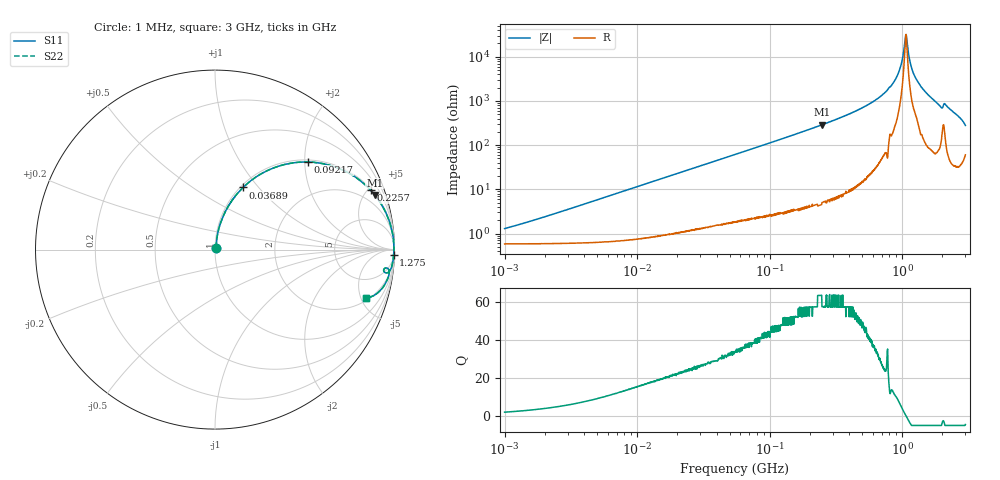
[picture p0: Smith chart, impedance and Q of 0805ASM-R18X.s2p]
!s-Parameter Generated by FASTRON Sdn. Bhd.
!FASTRON P/N : 0805ASM-R18X
!Keysight Technologies: E4991B_MY54100416_A.01.15
!Date: Fri Jun 19 14:50:46 2026
!Version  :Rev00  Fri Jun 19 14:50:46 2026
!Data & Calibration Information:
!Freq  S11  S21  S12  S22
!PortZ  Port1:50+j0  Port2:50+j0
!When reading reference impedance value at option line is always used.
! Remarks : This data is being provided solely for informational purposes.
# Hz S dB R 50
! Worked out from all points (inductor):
!   1601 points, 1 MHz to 3 GHz, reference 50 ohm
!   read as one part in series: L = 184 nH near 1.522 MHz
!   highest Q = 63.3 at 249.5 MHz (marker M1), where L = 185 nH
!   self-resonance near 1.065 GHz
!   S11 on the Smith chart (normalised r, x): 1 MHz: 1.01, +0.02; 36.89 MHz: 1.03, +0.83; 92.17 MHz: 1.05, +2.07; 225.7 MHz: 1.09, +5.20; 1.275 GHz: 10, -62; 3 GHz: 2.22, -5.47
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1000000  -37.80 62.6  -0.05 -0.7  -0.05 -0.7  -37.80 62.6
3804036  -27.10 79.6  -0.06 -2.5  -0.06 -2.5  -27.10 79.6
1.447069e7  -15.80 77.7  -0.19 -9.3  -0.19 -9.3  -15.80 77.7
3.688738e7  -8.41 65.7  -0.80 -22.3  -0.80 -22.3  -8.41 65.7
5.504702e7  -5.69 57.0  -1.52 -31.3  -1.52 -31.3  -5.69 57.0
9.216659e7  -2.97 43.4  -3.26 -45.2  -3.26 -45.2  -2.97 43.4
2.083556e8  -0.76 22.6  -8.32 -66.4  -8.32 -66.4  -0.76 22.6
2.257233e8  -0.65 20.9  -8.96 -68.1  -8.96 -68.1  -0.65 20.9
2.494827e8  -0.53 18.9  -9.80 -70.1  -9.80 -70.1  -0.53 18.9
5.284703e8  -0.10 7.4  -17.80 -81.3  -17.80 -81.3  -0.10 7.4
7.925923e8  -0.04 2.9  -25.90 -83.9  -25.90 -83.9  -0.04 2.9
9.395906e8  -0.03 1.3  -32.90 -81.3  -32.90 -81.3  -0.03 1.3
9.878038e8  -0.03 0.8  -37.00 -77.1  -37.00 -77.1  -0.03 0.8
1.0437e9  -0.03 0.2  -45.80 -53.1  -45.80 -53.1  -0.03 0.2
1.064802e9  -0.03 0.0  -50.00 -11.3  -50.00 -11.3  -0.03 0.0
1.097256e9  -0.03 -0.3  -44.90 55.8  -44.90 55.8  -0.03 -0.3
1.182785e9  -0.03 -1.1  -34.60 78.1  -34.60 78.1  -0.03 -1.1
1.274982e9  -0.04 -1.8  -30.00 80.2  -30.00 80.2  -0.04 -1.8
1.481494e9  -0.05 -3.4  -24.50 82.6  -24.50 82.6  -0.05 -3.4
1.912199e9  -0.18 -7.1  -18.10 76.9  -18.10 76.9  -0.18 -7.1
2.134733e9  -0.20 -6.8  -18.40 75.5  -18.40 75.5  -0.20 -6.8
3e9  -1.08 -17.9  -10.00 59.6  -10.00 59.6  -1.08 -17.9
